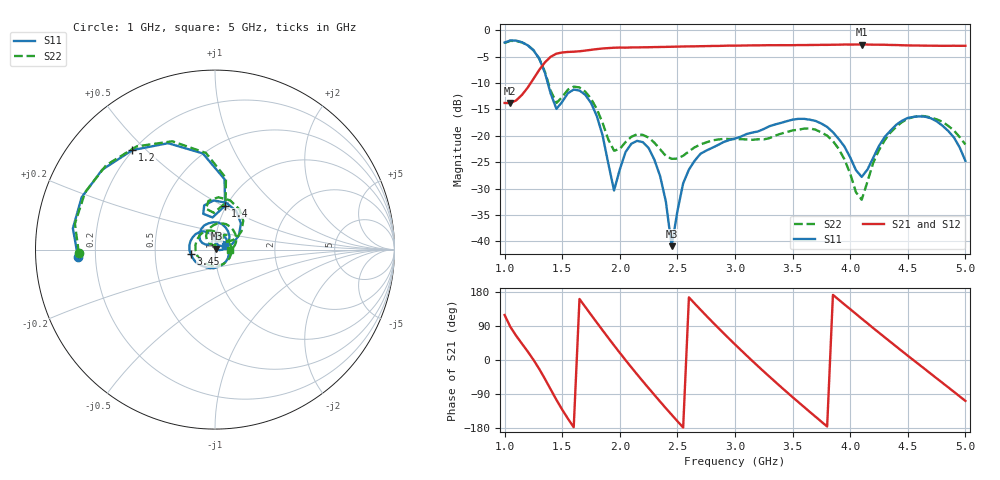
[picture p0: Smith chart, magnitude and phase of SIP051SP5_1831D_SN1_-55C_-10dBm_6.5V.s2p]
# GHz  S  dB  R  50
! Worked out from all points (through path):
!   81 points, 1 GHz to 5 GHz, reference 50 ohm
!   highest |S21| = -2.70 dB at 4.1 GHz (marker M1); lowest = -13.8 dB at 1.05 GHz (marker M2)
!   lowest |S11| = -40.9 dB at 2.45 GHz (marker M3), VSWR 1.02, Z = 50.8 + j0.445 ohm
!   |S11| at or under -10 dB: 1.375 GHz to end of sweep
!   |S22| runs from -32.1 to -2.0 dB; largest |S21 - S12| = 0.0025
!   S11 on the Smith chart (normalised r, x): 1 GHz: 0.13, -0.03; 1.2 GHz: 0.20, +0.45; 1.4 GHz: 0.99, +0.51; 3.45 GHz: 0.76, -0.04; 5 GHz: 1.11, +0.04
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1  -2.33 -177.0  -13.78 118.7  -13.78 118.8  -2.40 -178.7
1.05  -1.93 171.5  -13.81 87.4  -13.82 87.3  -2.01 169.5
1.2  -2.84 129.8  -10.88 22.6  -10.89 22.6  -2.83 127.2
1.4  -12.00 77.1  -5.02 -77.6  -5.02 -77.5  -11.46 77.3
1.55  -11.92 103.7  -4.11 -155.0  -4.12 -155.0  -11.24 97.7
1.7  -12.23 60.7  -3.85 140.2  -3.86 140.2  -11.63 58.6
1.95  -30.38 53.4  -3.31 38.5  -3.32 38.5  -22.84 43.7
2.05  -23.08 86.7  -3.29 -0.3  -3.29 -0.3  -21.20 61.5
2.2  -21.21 43.7  -3.23 -56.2  -3.24 -56.1  -19.84 42.2
2.35  -27.65 -0.8  -3.17 -109.8  -3.17 -109.8  -22.57 27.2
2.45  -40.93 29.2  -3.12 -144.4  -3.13 -144.5  -24.37 32.2
2.55  -29.02 85.0  -3.07 -178.2  -3.06 -178.2  -23.78 39.8
2.75  -22.82 19.4  -3.00 117.1  -3.01 117.1  -21.27 22.2
3  -20.54 -65.4  -2.92 41.1  -2.91 41.2  -20.61 -30.2
3.2  -19.17 -116.7  -2.86 -16.3  -2.86 -16.3  -20.66 -92.8
3.45  -17.24 -169.0  -2.83 -84.8  -2.82 -84.7  -19.28 -178.7
3.7  -17.19 141.1  -2.79 -150.0  -2.79 -150.0  -18.86 111.7
3.9  -20.60 107.0  -2.73 159.3  -2.73 159.3  -22.46 69.6
4.1  -27.80 125.5  -2.70 109.1  -2.68 109.1  -32.13 103.1
4.35  -19.02 140.5  -2.79 47.6  -2.80 47.6  -19.37 114.4
4.65  -16.39 83.4  -2.92 -24.3  -2.94 -24.4  -16.30 56.9
5  -24.76 19.5  -2.94 -107.9  -2.94 -108.0  -21.65 -1.8
